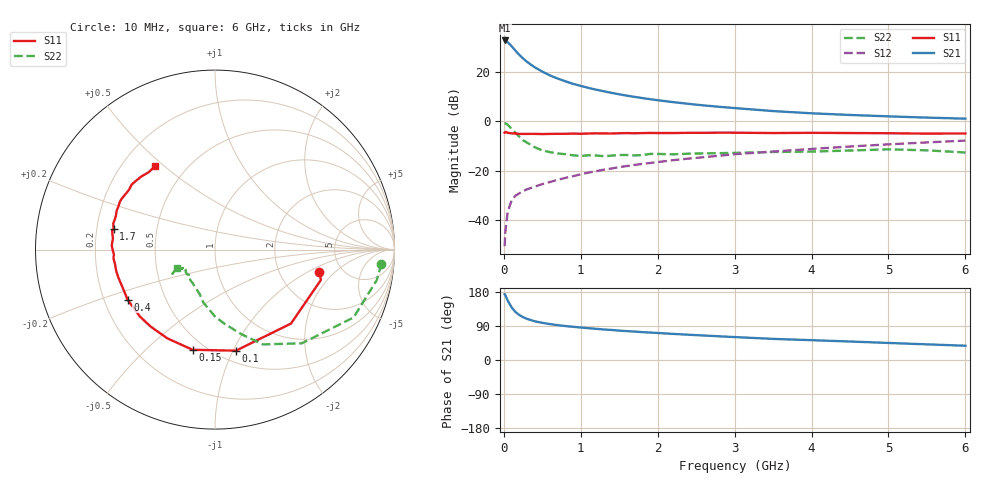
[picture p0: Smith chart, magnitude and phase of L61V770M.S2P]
!  INFINEON TECHNOLOGIES Small Signal Semiconductors
! BFR380L3 , Si-NPN RF-Transistor in TSLP-3-1
!  Vce=1.75 V,  Ic=70 mA
! Common Emitter S-Parameters:  07. March 2005
#  GHz  S  MA  R  50
! f  S11  S21  S12  S22
! GHz  Mag  Ang  Mag  Ang  Mag  Ang  Mag  Ang
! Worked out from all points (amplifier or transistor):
!   36 points, 10 MHz to 6 GHz, reference 50 ohm
!   highest |S21| = 32.8 dB at 10 MHz (marker M1)
!   |S21| within 3 dB of that: start of sweep to 119.5 MHz
!   unconditionally stable (mu >= 1): 1.199 GHz to 5.16 GHz
!   at 250 MHz: K = 0.53, MSG = 26.8 dB, |S12| = -28.2 dB
!   at 1.4 GHz: K = 1.02, MAG = 14.4 dB, |S12| = -19.0 dB
!   at 6 GHz: K = 0.98, MSG = 4.4 dB, |S12| = -7.7 dB
!   S11 on the Smith chart (normalised r, x): 10 MHz: 3.40, -1.29; 100 MHz: 0.61, -1.03; 150 MHz: 0.43, -0.71; 400 MHz: 0.30, -0.24; 1.7 GHz: 0.27, +0.10; 6 GHz: 0.34, +0.46
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0.01  0.5942 -11.9  43.56 173.6  0.003 75.2  0.9308 -4.9
0.02  0.6137 -16.0  43.34 170.8  0.006 81.3  0.9169 -10.7
0.05  0.5908 -44.2  40.32 156.9  0.0147 72.2  0.8597 -26.1
0.1  0.5751 -78.3  33.42 139.2  0.025 60.9  0.7116 -47.2
0.15  0.572 -102.6  27.17 126.9  0.0314 53.9  0.5917 -63.2
0.2  0.5612 -118.2  22.34 118.8  0.0352 52.2  0.4926 -72.8
0.25  0.559 -129.8  18.88 113.0  0.039 50.6  0.4158 -82.8
0.3  0.5604 -138.1  16.14 108.6  0.0424 51.0  0.3743 -89.8
0.4  0.5611 -150.2  12.53 102.2  0.0479 52.8  0.3021 -102.4
0.5  0.5564 -158.0  10.2 98.1  0.0541 55.2  0.2597 -109.6
0.6  0.5603 -163.6  8.529 94.7  0.0596 56.8  0.2396 -116.5
0.7  0.5629 -167.6  7.384 92.0  0.0661 59.2  0.225 -123.4
0.9  0.568 -175.2  5.774 87.6  0.0781 62.0  0.207 -133.7
1.1  0.5702 -179.9  4.779 83.9  0.0924 63.7  0.2076 -138.2
1.4  0.5718 173.8  3.79 79.3  0.1117 65.2  0.2036 -143.9
1.7  0.5771 168.3  3.143 75.0  0.132 65.7  0.206 -150.4
2.2  0.5833 161.2  2.464 68.9  0.1647 65.9  0.2164 -150.6
2.8  0.5934 153.2  1.981 62.5  0.203 65.7  0.2283 -154.7
3.5  0.5836 145.2  1.623 55.7  0.2463 63.4  0.2417 -152.7
4.5  0.5835 138.9  1.354 48.8  0.3114 61.2  0.2584 -151.4
5.5  0.5678 130.7  1.197 41.3  0.3771 57.1  0.2607 -151.4
6  0.5721 125.9  1.14 37.6  0.4105 54.7  0.2354 -154.9
